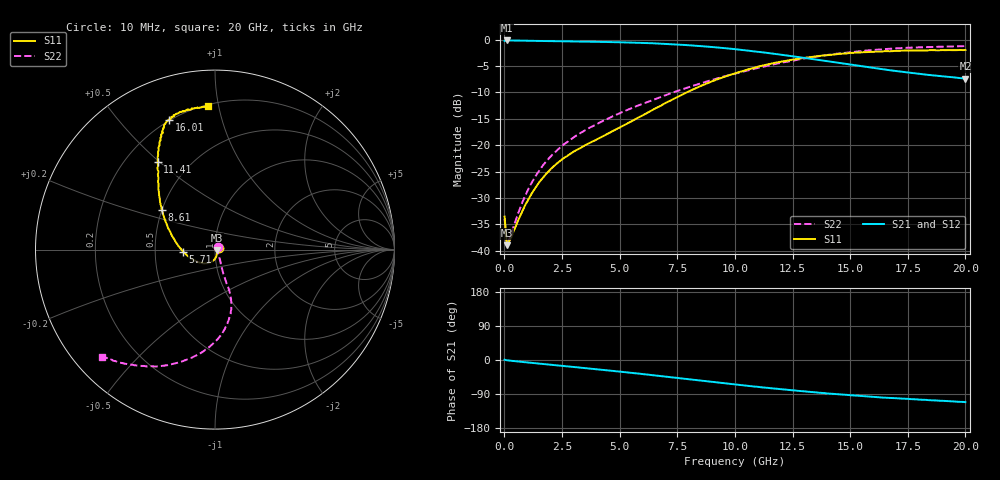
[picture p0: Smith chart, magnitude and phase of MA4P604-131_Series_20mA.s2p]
! AWR Design Environment (9226) Thu Aug 19 15:08:55 2021
! Document = '20mA'
! nPorts: 2, nXvals: 201
# GHz S DB R 50
!Freq DBS11 AngS11 DBS21 AngS21 DBS12 AngS12 DBS22 AngS22
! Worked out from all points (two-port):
!   201 points, 10 MHz to 20 GHz, reference 50 ohm
!   highest |S21| = -0.15 dB at 110 MHz (marker M1); lowest = -7.4 dB at 20 GHz (marker M2)
!   |S21| within 3 dB of the highest: start of sweep to 12.51 GHz
!   lowest |S11| = -39.0 dB at 110 MHz (marker M3), VSWR 1.02, Z = 51.1 - j0.21 ohm
!   |S11| at or under -10 dB: start of sweep to 7.906 GHz
!   |S22| runs from -39.1 to -1.2 dB; largest |S21 - S12| = 0.027
!   S11 on the Smith chart (normalised r, x): 10 MHz: 1.04, +0.01; 5.71 GHz: 0.70, -0.02; 8.61 GHz: 0.50, +0.26; 11.41 GHz: 0.33, +0.49; 16.01 GHz: 0.19, +0.69; 20 GHz: 0.21, +0.93
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0.01  -33.52 18.6  -0.22 0.8  -0.19 0.8  -33.96 36.2
0.11  -38.99 -10.5  -0.15 -0.8  -0.14 -0.8  -39.13 -11.3
0.31  -37.33 -31.0  -0.16 -2.1  -0.14 -2.1  -36.56 -31.3
0.81  -32.18 -61.8  -0.19 -5.3  -0.17 -5.2  -30.49 -52.6
1.11  -29.75 -72.9  -0.21 -7.2  -0.20 -7.0  -27.67 -58.3
1.41  -27.68 -81.7  -0.24 -9.0  -0.22 -8.8  -25.46 -61.9
1.81  -25.45 -91.9  -0.26 -11.4  -0.25 -11.1  -23.09 -65.2
2.21  -23.72 -101.6  -0.29 -13.7  -0.27 -13.4  -21.27 -67.6
2.61  -22.34 -110.9  -0.31 -16.1  -0.30 -15.7  -19.74 -69.3
3.41  -20.24 -128.2  -0.37 -20.9  -0.35 -20.4  -17.41 -70.6
4.71  -17.28 -156.2  -0.47 -28.8  -0.45 -28.2  -14.50 -71.1
5.71  -14.99 -176.3  -0.58 -35.2  -0.57 -34.4  -12.63 -70.7
6.71  -12.68 166.5  -0.73 -41.9  -0.72 -41.0  -10.99 -71.9
8.61  -8.62 143.0  -1.25 -54.9  -1.22 -53.6  -8.15 -78.3
10.01  -6.39 130.9  -1.80 -64.5  -1.74 -62.8  -6.44 -85.9
11.41  -4.70 123.4  -2.51 -73.4  -2.41 -71.8  -4.93 -96.1
13.41  -3.22 116.2  -3.70 -84.8  -3.55 -83.7  -3.29 -110.9
16.01  -2.29 109.6  -5.35 -97.3  -5.26 -96.5  -1.95 -126.8
16.71  -2.20 107.6  -5.78 -100.1  -5.74 -99.3  -1.72 -129.7
18.21  -2.04 103.0  -6.58 -104.9  -6.65 -104.7  -1.42 -134.3
19.51  -2.00 96.6  -7.15 -109.2  -7.33 -108.6  -1.28 -136.0
20  -1.95 92.7  -7.38 -111.2  -7.61 -110.0  -1.21 -136.4
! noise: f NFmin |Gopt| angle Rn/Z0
0.01  0  1  0  2e-20
2.21  0  1  0  2e-20
4.41  0  1  0  2e-20
6.61  0  1  0  2e-20
8.81  0  1  0  2e-20
11.11  0  1  0  2e-20
13.31  0  1  0  2e-20
15.51  0  1  0  2e-20
17.71  0  1  0  2e-20
20  0  1  0  2e-20
